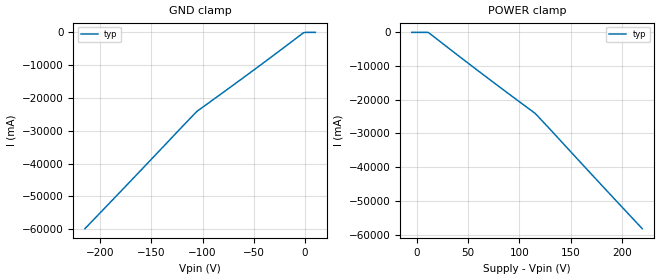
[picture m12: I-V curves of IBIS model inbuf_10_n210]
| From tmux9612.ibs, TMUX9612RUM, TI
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| inbuf_10_n210
[Model]   inbuf_10_n210
Model_type   Input
Vinl = 0.8
Vinh = 1.3
|   typ   min   max
C_comp   1.008417e-12   NA   NA
[Voltage Range]   10_210   NA   NA
[Temperature Range]   27   NA   NA
[Power Clamp Reference]   10_210   NA   NA
[GND Clamp Reference]   0   NA   NA
[GND Clamp]
|   Voltage   I(typ)   I(min)   I(max)
-215V     -59.87A    NA         NA
-105.9V   -24.18A    NA         NA
-1.364V   -75.61mA   NA         NA
10V       754.4nA    NA         NA
[POWER Clamp]
|   Voltage   I(typ)   I(min)   I(max)
-5V       1.035uA    NA         NA
10.91V    -4.166mA   NA         NA
115.5V    -24.05A    NA         NA
220V      -58.25A    NA         NA
